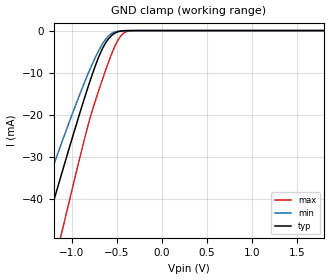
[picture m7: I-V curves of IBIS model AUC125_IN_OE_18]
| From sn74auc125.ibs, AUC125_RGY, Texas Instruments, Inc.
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[Model]   AUC125_IN_OE_18
Model_type  Input
Vinl=0.5775
Vinh=1.2675
| variable   typ   min   max
C_comp   2.58pF   2.10pF   3.00pF
[Temperature Range]   40   100   -40
| Ambient temperature   25   85   -40
[Voltage range]   1.8   1.65   1.95
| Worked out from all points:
|   GND clamp passes 1 mA (typ) near -0.55 V on its own axis
[GND Clamp]
| AUC125_IN_OE_18
|   Voltage   I(typ)   I(min)   I(max)
-3.6V     -222.6mA   -186.3mA   -267.8mA
-1.475V   -61.22mA   -48.92mA   -80.81mA
-1.43V    -57.84mA   -46.13mA   -76.8mA
-1.295V   -47.75mA   -37.84mA   -64.74mA
-1.1V     -33.37mA   -26.15mA   -47.31mA
-830mV    -14.32mA   -10.98mA   -23.64mA
-680mV    -5.364mA   -4.044mA   -13.09mA
-560mV    -1.272mA   -758.2uA   -5.827mA
-485mV    -290.6uA   -141.4uA   -2.305mA
-420mV    -55.81uA   -26.93uA   -608.5uA
-300mV    -1.501uA   -993.1nA   -11.88uA
1.8V      213.9pA    308.1pA    246.3pA
